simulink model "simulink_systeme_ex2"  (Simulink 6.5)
settings: Solver=ode45  StartTime=0.0  StopTime=0.2  RelTol=1e-3
PostLoadFcn:
  | simulink_systems_ex2
StartFcn:
  | simulink_systems_ex2
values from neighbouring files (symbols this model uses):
  Ti = 0.1    [simulink_systems_ex2.m]

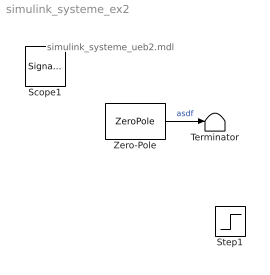
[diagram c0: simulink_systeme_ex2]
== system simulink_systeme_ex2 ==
  note: simulink_systeme_ueb2.mdl
  Terminator : Terminator
  Zero-Pole : ZeroPole  Zeros=[]  Poles=[0]  Gain=1/Ti
  Scope1 : SignalViewerScope  IOType=viewer  NumInputPorts=2  RefreshTime=0.035000
  Step1 : Step  IOType=siggen  SampleTime=0
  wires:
  Zero-Pole/1 -> Terminator/1  "asdf"
